FUNCTION_BLOCK Example22_stream //5x2 flyways 9 xbots (y axis feedback must be enabled) - StreamModeCtrl,WriteStream,ConfigFBStream,read feedback
VAR_INPUT
	Execute : BOOL;
END_VAR
VAR_OUTPUT
	Done : BOOL;
END_VAR
VAR_IN_OUT
	PM_Controller : PMControllerType;	// the planar motor controller to use
END_VAR
VAR
	PMC_StopXbots1 : PMC_StopXbots;
	xbotID_array78 : ARRAY[0..77] OF USINT;
	posx_array78 : ARRAY[0..77] OF REAL;
	posy_array78 : ARRAY[0..77] OF REAL;
	PMC_AutoDrivingMotion1 : PMC_AutoDrivingMotion;
	
	StmID_array8 : ARRAY[0..7] OF USINT;
	XbotID_array8 : ARRAY[0..7] OF USINT;
	FBmode_array8 : ARRAY[0..7] OF USINT;
	PMC_ConfigFBStream1 : PMC_ConfigFBStream;
	
	xbotID_array9 : ARRAY[0..8] OF USINT;
	stmID_array9 : ARRAY[0..8] OF USINT;
	stmAxis_array9 : ARRAY[0..8] OF USINT;
	PMC_StreamModeCtrl1 : PMC_StreamModeCtrl;
	
	read_y_pos : REAL;
	PMC_ReadStreamFeedback1 : PMC_ReadStreamFeedback;
	PMC_WriteStream1 : PMC_WriteStream;
	PMC_StreamModeCtrl2 : PMC_StreamModeCtrl;
		
	xindex : USINT;
	y_pos : REAL;
	
	following_error_mm : REAL;
END_VAR

//5x2 flyways 9 xbots (y axis feedback must be enabled) - StreamModeCtrl,WriteStream,ConfigFBStream,read feedback

IF Execute = FALSE THEN
	//reset streaming positions
	y_pos := 0;
	FOR xindex := 1 TO 10 DO
		PMC_WriteStream1(Enable := TRUE,StmID := xindex,AxisID := 1,Pos := 0,PM_Controller := PM_Controller);
		PMC_WriteStream1(Enable := TRUE,StmID := xindex,AxisID := 2,Pos := 0,PM_Controller := PM_Controller);
		PMC_WriteStream1(Enable := TRUE,StmID := xindex,AxisID := 3,Pos := 0,PM_Controller := PM_Controller);
		PMC_WriteStream1(Enable := TRUE,StmID := xindex,AxisID := 4,Pos := 0,PM_Controller := PM_Controller);
		PMC_WriteStream1(Enable := TRUE,StmID := xindex,AxisID := 5,Pos := 0,PM_Controller := PM_Controller);
		PMC_WriteStream1(Enable := TRUE,StmID := xindex,AxisID := 6,Pos := 0,PM_Controller := PM_Controller);
	END_FOR;
END_IF;

//Stop all xbots
PMC_StopXbots1(Execute := Execute,XbotID := 0,PM_Controller := PM_Controller);

//move all xbots to bottom of flyways
xbotID_array78[0] := 1; xbotID_array78[1] := 2; xbotID_array78[2] := 3; xbotID_array78[3] := 4; xbotID_array78[4] := 5; xbotID_array78[5] := 6; xbotID_array78[6] := 7; xbotID_array78[7] := 8; xbotID_array78[8] := 9;
posx_array78[0] := 0.06;posx_array78[1] := 0.18;posx_array78[2] := 0.30;posx_array78[3] := 0.42;posx_array78[4] := 0.54;posx_array78[5] := 0.66;posx_array78[6] := 0.78;posx_array78[7] := 0.90;posx_array78[8] := 1.02;
posy_array78[0] := 0.06;posy_array78[1] := 0.06;posy_array78[2] := 0.06;posy_array78[3] := 0.06;posy_array78[4] := 0.06;posy_array78[5] := 0.06;posy_array78[6] := 0.06;posy_array78[7] := 0.06;posy_array78[8] := 0.06;
PMC_AutoDrivingMotion1(Execute := PMC_StopXbots1.Done,nXbots := 9,RoutingType := 0,ZoneID := 0,XbotID := xbotID_array78,PosX := posx_array78,PosY := posy_array78,PM_Controller := PM_Controller);

//config feedback stream of xbot 1
StmID_array8[0] := 1;
XbotID_array8[0] := 5;
FBmode_array8[0] := 0;
PMC_ConfigFBStream1(Execute := PMC_AutoDrivingMotion1.Done,nStm := 1,StmID := StmID_array8,XbotID := XbotID_array8,FBMode := FBmode_array8,PM_Controller := PM_Controller);

//config streaming control for all 9 xbot's y axis
xbotID_array9[0] := 9;xbotID_array9[1] := 2;xbotID_array9[2] := 3;xbotID_array9[3] := 4;xbotID_array9[4] := 5;xbotID_array9[5] := 6;xbotID_array9[6] := 7;xbotID_array9[7] := 8;xbotID_array9[8] := 1;
stmID_array9[0] := 9; stmID_array9[1] := 2; stmID_array9[2] := 3; stmID_array9[3] := 4; stmID_array9[4] := 5; stmID_array9[5] := 6; stmID_array9[6] := 7; stmID_array9[7] := 8; stmID_array9[8] := 1; 
stmAxis_array9[0] :=2;stmAxis_array9[1] :=2;stmAxis_array9[2] :=2;stmAxis_array9[3] :=2;stmAxis_array9[4] :=2;stmAxis_array9[5] :=2;stmAxis_array9[6] :=2;stmAxis_array9[7] :=2;stmAxis_array9[8] :=2;
//xbotID_array9[0] := 1;xbotID_array9[1] := 2;xbotID_array9[2] := 3;xbotID_array9[3] := 4;xbotID_array9[4] := 5;xbotID_array9[5] := 6;xbotID_array9[6] := 7;xbotID_array9[7] := 8;xbotID_array9[8] := 9;
//stmID_array9[0] := 1; stmID_array9[1] := 2; stmID_array9[2] := 3; stmID_array9[3] := 4; stmID_array9[4] := 5; stmID_array9[5] := 6; stmID_array9[6] := 7; stmID_array9[7] := 8; stmID_array9[8] := 9; 
//stmAxis_array9[0] :=2;stmAxis_array9[1] :=2;stmAxis_array9[2] :=2;stmAxis_array9[3] :=2;stmAxis_array9[4] :=2;stmAxis_array9[5] :=2;stmAxis_array9[6] :=2;stmAxis_array9[7] :=2;stmAxis_array9[8] :=2;
PMC_StreamModeCtrl1(Execute := PMC_ConfigFBStream1.Done,Level := 1,nXbots := 9,XbotID := xbotID_array9,StmID := stmID_array9,StmAxis := stmAxis_array9,PM_Controller := PM_Controller);

//slowly move all xbots to top of flyways 
IF(PMC_StreamModeCtrl1.Done = TRUE AND y_pos < 0.36)THEN
	PMC_ReadStreamFeedback1(Enable := TRUE,StreamChannelID := 1,XBotAxisID := 2,FeedbackValue => read_y_pos,PM_Controller := PM_Controller);
	following_error_mm := 1000.0*((y_pos + 0.06) - read_y_pos);
	y_pos := y_pos + 0.00001;
	FOR xindex := 1 TO 10 DO
		PMC_WriteStream1(Enable := TRUE,StmID := xindex,AxisID := 2,Pos := y_pos,PM_Controller := PM_Controller);
	END_FOR; 
END_IF;
	
//stop streaming on all xbots
PMC_StreamModeCtrl2(Execute := PMC_StreamModeCtrl1.Done = TRUE AND y_pos >= 0.36,Level := 0,nXbots := 10,XbotID := xbotID_array9,StmID := stmID_array9,StmAxis := stmAxis_array9,PM_Controller := PM_Controller);

Done := PMC_StreamModeCtrl2.Done;

END_FUNCTION_BLOCK
